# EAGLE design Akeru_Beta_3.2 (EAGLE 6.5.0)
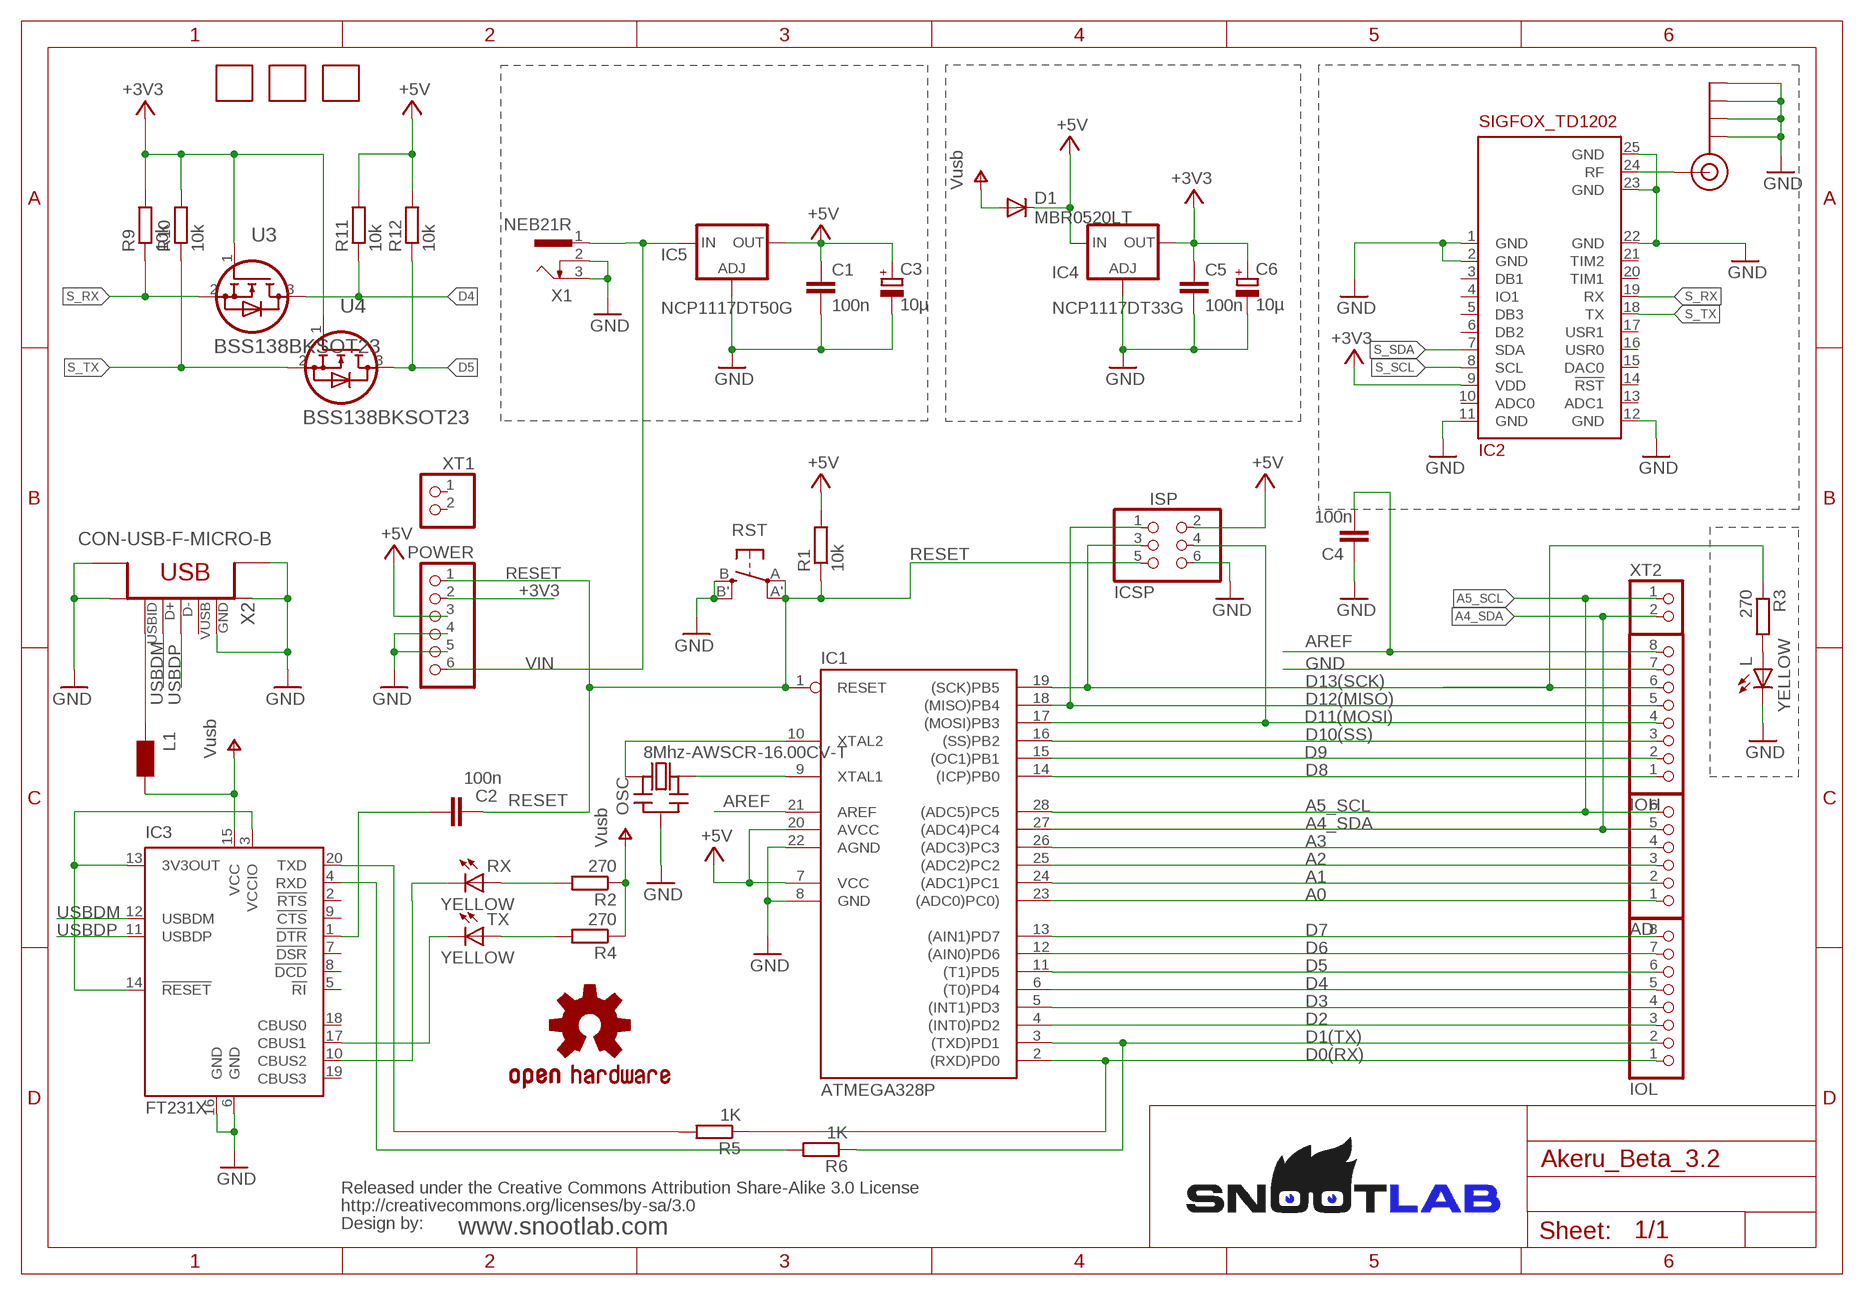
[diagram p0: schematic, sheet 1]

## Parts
AD  PINHD-1X6/STACK  [1X06_STACK]
C1  100n  C-EUC1206  [C1206]
C2  100n  C-EUC1206  [C1206]
C3  10µ  CPOL-EUC  [PANASONIC_C]
C4  100n  C-EUC1206  [C1206]
C5  100n  C-EUC1206  [C1206]
C6  10µ  CPOL-EUC  [PANASONIC_C]
D1  MBR0520LT  [SOD123]
IC1  ATMEGA328P  AT90S4433P  [DIL28-3]
IC2  SIGFOX_TD1202  [TD1202]
IC3  FT231X  [SSOP20]
IC4  NCP1117DT33G  LD117ADT33TR  [DPACK]
IC5  NCP1117DT50G  LD117ADT33TR  [DPACK]
IOH  PINHD-1X8/STACK  [1X08_STACK]
IOL  PINHD-1X8/STACK  [1X08_STACK]
ISP  ICSP  PINHD-2X3  [2X03]
J$1  SMA_EDGE  [SMA_EDGE]
L  YELLOW  LEDCHIPLED_1206  [CHIPLED_1206]
L1  WE-CBF_0805  [0805]
OSC  8Mhz-AWSCR-16.00CV-T  CERMOSCILL-AWCSR  [AWCSR]
POWER  PINHD-1X6/STACK  [1X06_STACK]
R1  10k  R-EU_R1206  [R1206]
R2  270  R-EU_R1206  [R1206]
R3  270  R-EU_R1206  [R1206]
R4  270  R-EU_M1206  [M1206]
R5  1K  R-EU_M1206  [M1206]
R6  1K  R-EU_M1206  [M1206]
R9  10k  R-EU_R1206  [R1206]
R10  10k  R-EU_R1206  [R1206]
R11  10k  R-EU_R1206  [R1206]
R12  10k  R-EU_R1206  [R1206]
RST  SPST_TACT-EVQQ2  [EVQ-Q2]
RX  YELLOW  LEDCHIPLED_1206  [CHIPLED_1206]
TX  YELLOW  LEDCHIPLED_1206  [CHIPLED_1206]
U3  BSS138BKSOT23  [SOT23]
U4  BSS138BKSOT23  [SOT23]
U$1  MARKER  [MARKER]
U$3  CREATIVE_COMMONS  [CREATIVE_COMMONS]
U$4  OSHW-LOGOL  [OSHW-LOGO-L]
U$7  MARKER  [MARKER]
U$8  MARKER  [MARKER]
X1  NEB21R  [NEB21R]
X2  CON-USB-F-MICRO-B  [DX4R005JJ2]
XT1  PINHD-1X2  [1X02_STACK]
XT2  PINHD-1X2  [1X02_STACK]

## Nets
+3V3: C5.1 C6.+ IC2.9(VDD) IC4.4(OUT) POWER.2 R9.2 R10.2 U3.1(G) U4.1(G)
+5V: C1.1 C3.+ D1.C IC1.7(VCC) IC1.20(AVCC) IC4.3(IN) IC5.4(OUT) ISP.2 POWER.3 R1.2 R11.2 R12.2
A0: AD.1 IC1.23((ADC0)PC0))
A1: AD.2 IC1.24((ADC1)PC1)
A2: AD.3 IC1.25((ADC2)PC2)
A3: AD.4 IC1.26((ADC3)PC3)
A4_SDA: AD.5 IC1.27((ADC4)PC4) XT2.2
A5_SCL: AD.6 IC1.28((ADC5)PC5) XT2.1
AREF: C4.2 IC1.21(AREF) IOH.8
D0(RX): IC1.2((RXD)PD0) IOL.1 R5.1
D1(TX): IC1.3((TXD)PD1) IOL.2 R6.1
D2: IC1.4((INT0)PD2) IOL.3
D3: IC1.5((INT1)PD3) IOL.4
D4: IC1.6((T0)PD4) IOL.5 R11.1 U3.3(D)
D5: IC1.11((T1)PD5) IOL.6 R12.1 U4.3(D)
D6: IC1.12((AIN0)PD6) IOL.7
D7: IC1.13((AIN1)PD7) IOL.8
D8: IC1.14((ICP)PB0) IOH.1
D9: IC1.15((OC1)PB1) IOH.2
D10(SS): IC1.16((SS)PB2) IOH.3
D11(MOSI): IC1.17((MOSI)PB3) IOH.4 ISP.4
D12(MISO): IC1.18((MISO)PB4) IOH.5 ISP.1
D13(SCK): IC1.19((SCK)PB5) IOH.6 ISP.3 R3.1
GND: C1.2 C3.- C4.1 C5.2 C6.- IC1.8(GND) IC1.22(AGND) IC2.1(GND) IC2.2(GND) IC2.11(GND) IC2.12(GND) IC2.22(GND) IC2.23(GND) IC2.25(GND) IC3.6(GND) IC3.16(GND) IC4.1(ADJ) IC5.1(ADJ) IOH.7 ISP.6 J$1.GND@0(GND) J$1.GND@1(GND) J$1.GND@2(GND) J$1.GND@3(GND) L.C OSC.2(GND) POWER.4 POWER.5 RST.B'(S1) RST.B(S) X1.2 X1.3 X2.BODY@1(BODY1) X2.BODY@2(BODY2) X2.BODY@3(BODY3) X2.BODY@6(BODY6) X2.P5(GND)
N$1: C2.2 IC3.1(!DTR)
N$2: L.A R3.2
N$3: IC2.24(RF) J$1.SIG(SIGNAL)
N$4: IC3.3(VCCIO) IC3.13(3V3OUT) IC3.14(!RESET)
N$5: IC3.17(CBUS1) TX.C
N$6: L1.1 X2.P4(USBID)
N$9: IC3.10(CBUS2) RX.C
N$10: R2.2 RX.A
N$11: R4.2 TX.A
N$12: IC3.20(TXD) R5.2
N$13: IC3.4(RXD) R6.2
RESET: C2.1 IC1.1(RESET) ISP.5 POWER.1 R1.1 RST.A'(P1) RST.A(P)
S_RX: IC2.19(RX) R9.1 U3.2(S)
S_SCL: IC2.8(SCL)
S_SDA: IC2.7(SDA)
S_TX: IC2.18(TX) R10.1 U4.2(S)
USBDM: IC3.12(USBDM) X2.P3(D+)
USBDP: IC3.11(USBDP) X2.P2(D-)
V+: D1.A IC3.15(VCC) L1.2 R2.1 R4.1 ; supply symbol labelled Vusb
VIN: IC5.3(IN) POWER.6 X1.1
XTAL1: IC1.9(XTAL1) OSC.3(OUT)
XTAL2: IC1.10(XTAL2) OSC.1(IN)
Unconnected: IC2.3(DB1) IC2.4(IO1) IC2.5(DB3) IC2.6(DB2) IC2.10(ADC0) IC2.13(ADC1) IC2.14(!RST) IC2.15(DAC0) IC2.16(USR0) IC2.17(USR1) IC2.20(TIM1) IC2.21(TIM2) IC3.2(!RTS) IC3.5(!RI) IC3.7(!DSR) IC3.8(!DCD) IC3.9(!CTS) IC3.18(CBUS0) IC3.19(CBUS3) X2.P1(VUSB) XT1.1 XT1.2

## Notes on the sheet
- www.snootlab.com

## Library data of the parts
AD POWER = SnootLib:PINHD-1X6: PIN HEADER
C1 C5 = rcl:C-EU: CAPACITOR, European symbol
C2 C4 = SmartPrj:C-EU: CAPACITOR, European symbol
C3 C6 = rcl:CPOL-EU: POLARIZED CAPACITOR, European symbol
D1 = diode:MBR0520LT: SCHOTTKY BARRIER RECTIFIER
IC1 = atmel:AT90S4433: MICROCONTROLLER 4 Kbytes FLASH 128 bytes SRAM 256 bytes EEPROM UART 6-channel 10 bit ADC; OC_FARNELL: unknown; OC_NEWARK: unknown
IC2 = SnootLib:SIGFOX_TD1202: Telecom Design SIGFOX TD1202 - 868MHz
IC3 = ftdichip:FT231X
IC4 IC5 = v-reg:LD117A?*: Low drop fixed and adjustable positive voltage regulators 1 A Source: http://www.st.com/stonline/products/literature/ds/7194/ld1117axx.pdf
IOH IOL = SnootLib:PINHD-1X8: PIN HEADER
ISP = pinhead:PINHD-2X3: PIN HEADER
J$1 = SnootLib:SMA_EDGE: SMA Antenna Connector End launch SMA connector. The paste layer has been removed so that the connector can be hand soldered onto the board after reflow.
L RX TX = led:LED: LED
L1 = wuerth-elektronik:WE-CBF: SMD EMI Suppression Ferrite Beads
OSC = adafruit:CERMOSCILL: Ceramic oscillator with built in capacitors such as ZTT-12MHz http://www.ladyada.net/library/eagle
R1-R6 R9-R12 = rcl:R-EU_: RESISTOR, European symbol
RST = adafruit:SPST_TACT: SMT 6mm switch, EVQQ2 series http://www.ladyada.net/library/eagle
U3 U4 = SnootLib:BSS138BK: N-channel Trench MOSFET
U$1 U$7 U$8 = lib:MARKER
U$3 = SnootLib:CREATIVE_COMMONS
U$4 = SparkFun:OSHW-LOGO: Open Source Hardware Logo This logo indicates the piece of hardware it is found on incorporates a OSHW license and/or adheres to the definition of open source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
X1 = SnootLib:NEB21R: Netzgeräte-Einbaukupplung abgewinkelte Ausführung mit Öffner Source: http://www.lumberg.com/Produkte/PDFs/NEB21R.pdf
X2 = SnootLib:CON-USB-F: USB Female connector
XT1 XT2 = SnootLib:PINHD-1X2

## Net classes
0 default: width 0.254 mm, drill 0.305 mm, clearance 0.152 mm
2 gnd: width 0.305 mm, drill 0.508 mm, clearance 0.152 mm
3 usbvcc: width 0.508 mm, drill 0.508 mm, clearance 0.152 mm

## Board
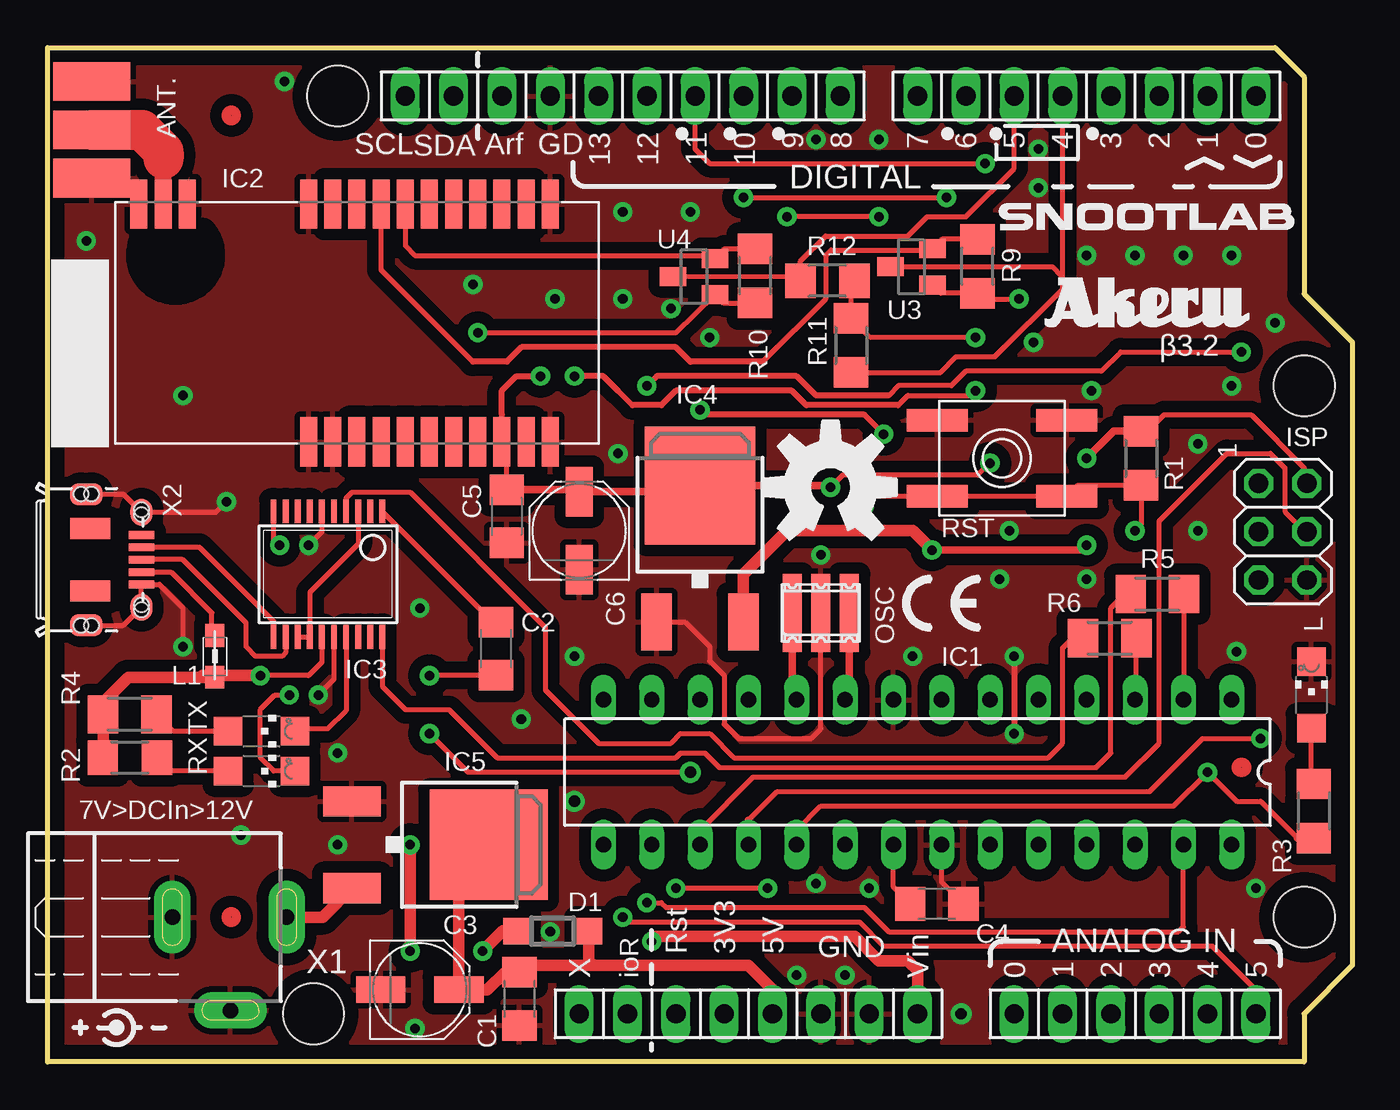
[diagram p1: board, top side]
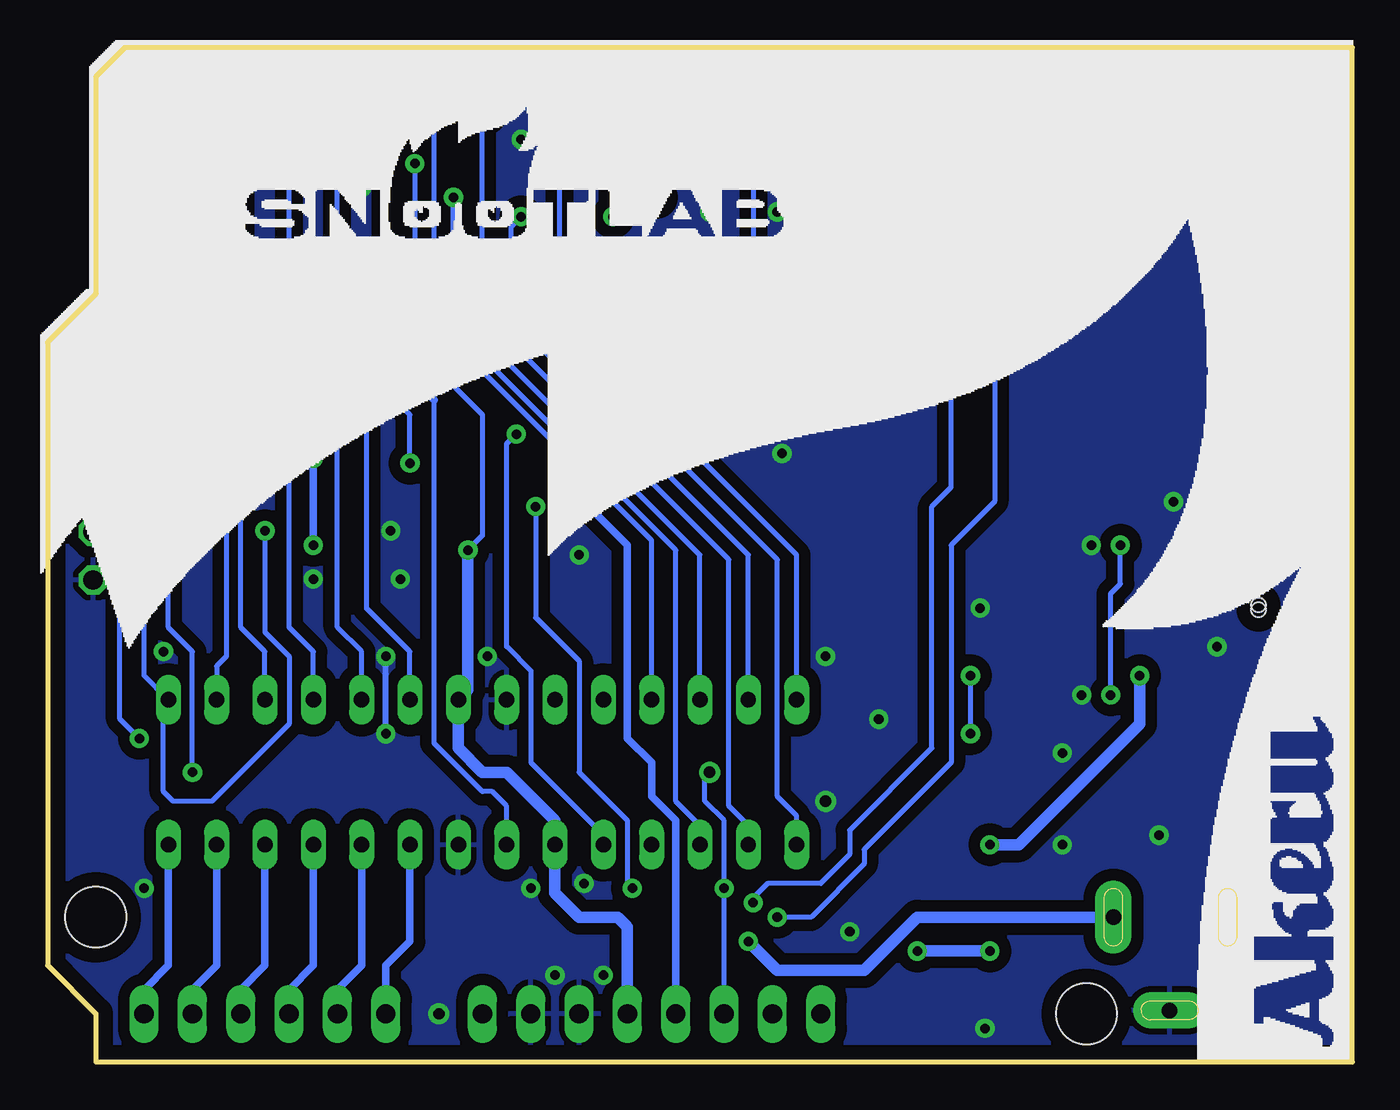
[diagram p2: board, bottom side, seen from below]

Size 68.58 x 53.34 mm. Coordinates in mm from the lower left corner, seen from the top.
Outline: 0,53.34 64.52,53.34 66.04,51.82 66.04,40.39 68.58,37.85 68.58,5.08 66.04,2.54 66.04,0 0,0 0,53.34
Copper layers (1*16): Top 0.035mm / dielectric 1.5mm / Bottom 0.035mm
Design rules "default *": minimum track width 8mil, minimum drill 12mil, track to track 6mil, track to pad 6mil, pad to pad 6mil, via to via 6mil, smd to smd 6mil, copper to edge 30mil, drill to drill 12mil, minimum pad ring 10mil, minimum via ring 10mil, stop-mask expansion 4mil, vias tented up to drill 30mil, thermal gap 12mil
Holes 3.2 mm at 66.04,35.55 66.04,7.61 15.24,50.79 13.97,2.53

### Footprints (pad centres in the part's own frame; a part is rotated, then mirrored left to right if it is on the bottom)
1X06_STACK = drill 1.016 long: 1 -6.35,0; 2 -3.81,0; 3 -1.27,0; 4 1.27,0; 5 3.81,0; 6 6.35,0
C1206 = smd 1.6 x 1.8: 1 -1.4,0; 2 1.4,0
PANASONIC_C = smd 2.6 x 1.4: + 2.05,0; - -2.05,0
SOD123 = smd 1.4 x 1.4: A 1.9,0; C -1.9,0
DIL28-3 = drill 0.813 long: 1 -16.51,-3.81; 2 -13.97,-3.81; 3 -11.43,-3.81; 4 -8.89,-3.81; 5 -6.35,-3.81; 6 -3.81,-3.81; 7 -1.27,-3.81; 8 1.27,-3.81; 9 3.81,-3.81; 10 6.35,-3.81; 11 8.89,-3.81; 12 11.43,-3.81; 13 13.97,-3.81; 14 16.51,-3.81; 15 16.51,3.81; 16 13.97,3.81; 17 11.43,3.81; 18 8.89,3.81; 19 6.35,3.81; 20 3.81,3.81; 21 1.27,3.81; 22 -1.27,3.81; 23 -3.81,3.81; 24 -6.35,3.81; 25 -8.89,3.81; 26 -11.43,3.81; 27 -13.97,3.81; 28 -16.51,3.81
TD1202 = smd 0.89 x 2.6: 1 -2.54,-6.25; 2 -1.27,-6.25; 3 0,-6.25; 4 1.27,-6.25; 5 2.54,-6.25; 6 3.81,-6.25; 7 5.08,-6.25; 8 6.35,-6.25; 9 7.62,-6.25; 10 8.89,-6.25; 11 10.16,-6.25; 12 10.16,6.25; 13 8.89,6.25; 14 7.62,6.25; 15 6.35,6.25; 16 5.08,6.25; 17 3.81,6.25; 18 2.54,6.25; 19 1.27,6.25; 20 0,6.25; 21 -1.27,6.25; 22 -2.54,6.25; 23 -8.92,6.25; 24 -10.19,6.25; 25 -11.46,6.25
SSOP20 = smd 0.305 x 1.245: 1 -2.857,-3.302; 2 -2.222,-3.302; 3 -1.587,-3.302; 4 -0.952,-3.302; 5 -0.317,-3.302; 6 0.318,-3.302; 7 0.953,-3.302; 8 1.588,-3.302; 9 2.223,-3.302; 10 2.858,-3.302; 11 2.858,3.302; 12 2.223,3.302; 13 1.588,3.302; 14 0.953,3.302; 15 0.318,3.302; 16 -0.317,3.302; 17 -0.952,3.302; 18 -1.587,3.302; 19 -2.222,3.302; 20 -2.857,3.302
DPACK = smd 1.6 x 3: 1 -2.28,-4.8; 3 2.28,-4.8 | smd 5.8 x 6.2: 4 0,2.38
1X08_STACK = drill 1.016 long: 1 -8.89,0; 2 -6.35,0; 3 -3.81,0; 4 -1.27,0; 5 1.27,0; 6 3.81,0; 7 6.35,0; 8 8.89,0
2X03 = drill 1.016 octagon: 1 -2.54,-1.27; 2 -2.54,1.27; 3 0,-1.27; 4 0,1.27; 5 2.54,-1.27; 6 2.54,1.27
SMA_EDGE = smd 2.032 x 4.064: GND@0 0,0; GND@1 5.08,0; SIG 2.54,0 | smd 2.032 x 4.064 bottom: GND@2 0,0; GND@3 5.08,0
CHIPLED_1206 = smd 1.5 x 1.5: A 0,-1.75; C 0,1.75
0805 = smd 1.2 x 1: 1 -1.1,0; 2 1.1,0
AWCSR = smd 1 x 4.1: 1 -1.5,0; 2 0,0; 3 1.5,0
R1206 = smd 1.6 x 1.803: 1 -1.422,0; 2 1.422,0
M1206 = smd 1.6 x 2: 1 -1.4,0; 2 1.4,0
EVQ-Q2 = smd 3.2 x 1.2: A -3.4,-2; A' 3.4,-2; B -3.4,2; B' 3.4,2
SOT23 = smd 1 x 1.4: 1 -0.95,-1.1; 2 0.95,-1.1; 3 0,1.1
NEB21R = drill 0.813 pad 1.93 long: 1 0,7.35; 2 4.9,4.4; 3 0,1.35
DX4R005JJ2 = smd 1.4 x 1.15: BODY@1 -2.5,2.9; BODY@2 2.5,2.9 | smd 1.15 x 1.7: BODY@3 3.45,0; BODY@6 -3.45,0 | smd 1.1 x 2.1: BODY@4 1.65,0.2; BODY@5 -1.65,0.2 | smd 0.4 x 1.35: P1 -1.3,2.9; P2 -0.65,2.9; P3 0,2.9; P4 0.65,2.9; P5 1.3,2.9 | hole 0.75: -2.625,2.9; -2.375,2.9; 2.375,2.9; 2.625,2.9; -3.45,0.275; -3.45,-0.275; 3.45,0.275; 3.45,-0.275
1X02_STACK = drill 1.016 long: 1 -1.27,0; 2 1.27,0

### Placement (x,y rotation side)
AD  57.15,2.53 0 top
C1  24.8,3.33 270 top
C2  23.57,21.73 90 top
C3  19.56,3.8 0 top
C4  46.74,8.31 180 top
C5  24.13,28.7 270 top
C6  27.94,27.93 90 top
D1  26.55,6.88 180 top
IC1  45.72,15.23 180 top
IC2  16.26,38.86 0 top
IC3  14.74,25.65 180 top
IC4  34.29,27.93 0 top
IC5  20.8,11.42 270 top
IOH  32.77,50.79 180 top
IOL  54.61,50.79 180 top
ISP  64.91,27.88 270 top
J$1  2.32,46.48 90 top
L  66.42,19.3 0 top
L1  8.8,21.33 270 top
OSC  40.64,23.62 0 top
POWER  39.37,2.53 0 top
R1  57.47,31.74 90 top
R2  4.32,16 0 top
R3  66.55,13.2 90 top
R4  4.32,18.28 0 top
R5  58.33,24.6 180 top
R6  55.82,22.28 180 top
R9  48.87,41.84 270 top
R10  37.18,41.33 270 top
R11  42.23,37.68 90 top
R12  40.99,41.08 0 top
RST  50.17,31.74 0 top
RX  11.24,15.3 270 top
TX  11.24,17.39 270 top
U3  45.41,41.81 90 top
U4  33.98,41.3 90 top
U$1  62.74,15.49 0 top
U$2  [CE3.08X4.13_TOP]  47.76,24.12 0 top
U$3  not placed on the board
U$4  41.15,30.22 0 top
U$5  [LOGO_SNOOT_FULL_H5]  not placed on the board
U$7  9.66,7.61 0 top
U$8  9.66,49.78 0 top
U$9  [LOGO_SNOOT_TXT_H1.7]  49.96,43.66 0 top
X1  5.21,7.61 270 top
X2  2.04,26.41 270 top
XT1  29.21,2.53 0 top
XT2  20.07,50.79 0 top

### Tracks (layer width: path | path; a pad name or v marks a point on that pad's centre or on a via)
+3V3  (via drill 0.5, 0.5 pad 0.25)
  Top 0.254: v22.61,38.35 33,38.35 U4.1 35.52,39.91 R10.2 | v49.53,31.49 48.9,30.85 41.79,30.85 v41.15,30.22 | C5.1 24.13,32.35 IC2.9 23.88,34.03 | U3.1 46.95,40.42 R9.2 49.37,40.13 v51.06,40.13
  Top 0.305: 23.88,34.03 23.88,35.3 24.64,36.06 v25.91,36.06
  Top 0.406: C5.1 27.83,30.1 C6.+ 33.96,29.98 IC4.4 41.06,30.31 v41.15,30.22
  Bottom 0.254: v49.53,31.49 49.53,34.03 50.04,34.54 50.04,39.11 v51.06,40.13
  Bottom 0.305: v25.91,36.06 25.91,36.57 24.13,38.35 v22.61,38.35
  Bottom 0.406: POWER.2 35.56,12.69 36.83,13.96 36.83,15.74 38.1,17.01 38.1,27.17 v41.15,30.22
+5V  (via drill 0.5, 0.5 pad 0.25)
  Top 0.254: R1.2 57.81,33.17 58.68,34.03 63.25,34.03 66.04,31.24 66.04,30.56 ISP.2 | R12.2 42.23,40.89 R11.2 43.24,38.09 v48.77,38.09
  Top 0.406: 57.41,33.23 R1.2 56.04,33.17 v54.61,31.74 | v54.61,27.17 54.36,26.92 v46.49,26.92
  Top 0.61: 28.71,5.07 25.15,5.07 C1.1 24.04,4.73 23.12,3.8 C3.+ 21.61,11.42 IC5.4 | 28.71,5.07 36.83,5.07 38.1,3.8 POWER.3 | IC4.3 36.57,25.64 38.87,27.93 45.47,27.93 v46.49,26.92 | D1.C 28.45,5.33 28.71,5.07
  Bottom 0.254: v48.77,38.09 48.77,37.08 45.72,34.03 45.72,27.68 v46.49,26.92
  Bottom 0.406: v54.61,31.74 v54.61,27.17 54.61,26.92
  Bottom 0.61: POWER.3 38.1,7.11 38.61,7.61 40.64,7.61 41.91,8.88 IC1.20 41.91,12.69 44.45,15.23 45.72,15.23 46.99,16.5 IC1.7 46.49,19.55 v46.49,26.92
A0
  Bottom 0.406: AD.1 50.8,5.07 49.53,6.34 IC1.23
A1
  Bottom 0.406: AD.2 53.34,3.8 52.07,5.07 IC1.24
A2
  Bottom 0.406: AD.3 55.88,3.8 54.61,5.07 IC1.25
A3
  Bottom 0.406: AD.4 58.42,3.8 57.15,5.07 IC1.26
A4_SDA  (via drill 0.5 pad 0.25)
  Top 0.254: v31.5,8.38 32.26,8.38 32.52,8.12 42.93,8.12 44.2,6.85 59.44,6.85 59.69,7.11 IC1.27
  Bottom 0.254: XT2.2 21.09,50.54 21.09,30.22 22.1,29.2 22.1,16.5 26.42,12.19 26.42,10.92 27.94,9.39 30.74,9.39 31.5,8.63 v31.5,8.38
  Bottom 0.406: AD.5 60.96,3.8 59.69,5.07 IC1.27
A5_SCL  (via drill 0.5 pad 0.25)
  Top 0.254: v30.23,7.61 30.48,7.36 42.68,7.36 43.95,6.09 61.22,6.09 63.5,3.8 AD.6
  Bottom 0.254: XT2.1 18.8,29.46 21.09,27.17 21.09,15.74 25.66,11.17 25.66,10.41 28.45,7.61 v30.23,7.61
  Bottom 0.406: IC1.28 62.23,5.07 63.5,3.8 AD.6
AREF  (via drill 0.5 pad 0.25)
  Top 0.254: 29.98,35.3 30.74,34.54 | 44.71,34.54 45.22,35.05 48.52,35.05 v48.77,35.3 | C4.2 44.45,9.2 IC1.21
  Top 0.305: 29.98,35.3 29.21,36.06 v27.69,36.06 | 44.71,34.54 39.88,34.54 39.12,35.3 33.02,35.3 32.26,34.54 30.74,34.54
  Bottom 0.254: 48.26,34.79 48.26,16.76 45.72,14.22 45.22,14.22 44.45,13.46 IC1.21
  Bottom 0.305: v27.69,36.06 23.88,39.87 IOH.8
  Bottom 0.406: v48.77,35.3 48.26,34.79
D0(RX)
  Top 0.254: 59.73,19.14 R5.1
  Top 0.406: IC1.2 59.66,19.08 59.73,19.14
  Bottom 0.254: IOL.1 63.5,40.13 59.19,35.81 59.19,21.33 59.69,20.82 IC1.2
D1(TX)
  Top 0.254: 57.22,19.24 R6.1
  Top 0.406: IC1.3 57.09,19.11 57.22,19.24
  Bottom 0.254: IC1.3 57.15,21.58 58.42,22.85 58.42,36.82 60.96,39.36 IOL.2
D2
  Bottom 0.254: IC1.4 54.61,21.58 55.88,22.85 55.88,36.82 58.42,39.36 IOL.3
D3
  Bottom 0.254: IC1.5 52.07,21.58 53.34,22.85 53.34,36.82 55.88,39.36 IOL.4
D4
  Top 0.254: 53.34,41.4 53.34,40.63 49.79,37.08 47.76,37.08 46.94,36.26 R11.1 | 53.34,41.4 IOL.5 | 53.34,41.4 53.28,41.33 52.8,41.81 U3.3
  Bottom 0.254: IC1.6 49.53,21.58 51.82,23.87 51.82,36.57 53.34,38.09 IOL.5
D5
  Top 0.254: 50.8,47.24 IOL.6 50.8,46.98 48.26,44.44 46.23,44.44 45.22,43.43 40.9,43.43 39.57,42.1 R12.1 39.32,41.33 U4.3
  Bottom 0.254: IC1.11 36.83,27.43 50.8,41.4 IOL.6
D6
  Bottom 0.254: IC1.12 34.29,26.66 48.26,40.63 IOL.7
D7
  Bottom 0.254: IC1.13 31.75,26.66 45.72,40.63 IOL.8
D8
  Bottom 0.254: IOH.1 41.66,46.98 | IC1.14 29.21,26.66 41.66,39.11 41.66,46.73
  Bottom 0.406: 41.66,46.98 41.66,46.73
D9  (via drill 0.5 pad 0.25)
  Top 0.254: v43.69,44.44 v38.87,44.44
  Bottom 0.254: IC1.15 29.21,12.95 30.23,13.96 30.23,26.41 44.2,40.38 44.2,43.94 v43.69,44.44 | v38.87,44.44 38.87,50.54
  Bottom 0.406: 38.87,50.54 IOH.2
D10(SS)  (via drill 0.5 pad 0.25)
  Top 0.254: v36.58,45.46 v47.25,45.46
  Bottom 0.254: IC1.16 31.75,12.44 32.77,13.46 32.77,26.41 47.25,40.89 v47.25,45.46 | v36.58,45.46 IOH.3
D11(MOSI)  (via drill 0.5)
  Top 0.254: 34.29,11.68 34.29,12.19 37.09,14.98 56.65,14.98 58.42,16.76 58.42,28.44 61.98,32 64.27,32 65.03,31.24 65.03,28.95 66.09,27.88 ISP.4 | v49.28,47.24 34.8,47.24 34.04,48 IOH.4
  Top 0.406: IC1.17 34.29,11.68
  Bottom 0.254: IC1.17 34.29,12.44 35.56,13.71 35.56,26.92 49.28,40.63 v49.28,47.24
D12(MISO)  (via drill 0.5, 0.5 pad 0.25)
  Top 0.254: 36.83,12.69 38.36,14.22 57.92,14.22 60.71,17.01 v63.76,17.01 | v62.74,37.33 56.39,37.33 55.38,36.32 48.26,36.32 47.5,35.55 44.71,35.55 44.2,35.05
  Top 0.305: 44.2,35.05 40.39,35.05 39.37,36.06 32.01,36.06 v31.5,35.55
  Top 0.406: IC1.18 36.83,12.69
  Bottom 0.254: IOH.5 v31.5,35.55 | v62.74,37.33 63.25,36.82 63.25,30.82 ISP.1 64.77,29.29 64.77,18.03 v63.76,17.01
D13(SCK)  (via drill 0.5 pad 0.25)
  Top 0.254: 42.93,34.03 v43.95,33.01 | IC1.19 39.37,12.19 40.64,13.46 59.19,13.46 v60.96,15.23 62.49,13.71 63.76,13.71 65.69,11.78
  Top 0.305: 42.93,34.03 34.55,34.03 v34.29,34.28
  Top 0.406: 65.69,11.78 R3.1
  Bottom 0.254: v60.96,15.23 60.96,21.58 62.23,22.85 62.23,27.93 63.59,27.93 ISP.3 | IOH.6 28.96,34.54 | 39.37,11.93 43.18,15.74 43.18,20.57 44.45,21.84 44.45,32.51 v43.95,33.01
  Bottom 0.305: 28.96,34.54 28.96,34.28 29.47,33.78 33.79,33.78 v34.29,34.28
  Bottom 0.406: 39.37,11.93 IC1.19
GND  (via drill 0.5 pad 0.25, 0.6 pad 0.25)
  Top 0.254: 15.05,22.66 IC3.16 15.05,20.12 v14.23,19.3 | IC4.1 33.51,23.13 34.8,21.84 34.8,21.08 35.56,20.31 35.56,17.77 36.33,17.01 40.14,17.01 40.64,17.52 OSC.2 | C4.1 46.99,9.46 IC1.22 | IC3.6 14.42,27.87 v13.72,27.17 | v7.12,21.84 7.12,23.87 5.88,25.11 X2.P5 X2.BODY@2 3.99,22.96 X2.BODY@3 | X2.BODY@6 3.99,29.86 X2.BODY@1 8.85,28.91 v9.4,29.46
  Top 0.305: 50.8,21.08 v50.8,17.27
  Bottom 0.305: v50.8,17.27 v50.8,21.33
  other vias: 27.69,21.33 7.12,35.05 10.16,11.93 26.42,6.85 27.69,13.71 45.47,21.33 50.04,25.39 48.01,2.53 63.5,9.14 64.52,38.86 62.23,35.55 60.46,27.93 32.77,39.62 15.24,16.25 19.31,1.77 50.55,27.93 26.67,40.13 22.36,40.89 60.46,32.51 54.87,35.3 29.98,32 40.64,26.66 39.37,4.57 52.07,48 51.82,37.84 52.07,45.97 54.61,42.41 57.15,42.41 59.69,42.41 41.91,4.57 43.18,9.14 40.39,9.39 34.8,38.09 62.49,21.58 54.61,25.39 62.23,42.41 15.24,11.42 43.69,48.51 40.39,48.51 30.23,44.7 30.23,40.13 33.79,44.7 2.04,43.17 12.45,51.56 24.9,18.03 19.56,23.87
  pour Bottom (isolate 0.61, rank 2): -1.52,52.7 67.69,52.7 67.95,52.44 67.95,0.63 -1.52,0.63
  pour Top (isolate 0.61, rank 2): -1.9,52.7 68.33,52.57 68.33,0.5 -1.9,0.63
N$1
  Top 0.254: IC3.1 23.41,23.13 C2.2
N$2
  Top 0.254: 66.42,14.75 L.A
  Top 0.406: R3.2 66.42,14.75
N$3
  Top 0.9: IC2.24 6.07,47.46 6.1,47.49
  Top 2.1: J$1.SIG 4.96,49.02 6.1,47.87 6.1,47.49
N$4
  Top 0.254: IC3.13 IC3.14 13.78,24.69 16.32,27.23 IC3.3
N$5
  Top 0.254: 13.63,17.52 TX.C 13.12,17.52 14.74,17.52 15.69,18.47 IC3.17
N$6
  Top 0.254: X2.P4 6.5,25.76 8.64,23.62 8.64,22.43 L1.1
N$9  (via drill 0.5)
  Top 0.254: 13.56,14.73 RX.C 11.88,15.3 11.18,16 11.18,18.54 11.94,19.3 v12.7,19.3 | v12.2,27.17 11.88,27.49 IC3.10
  Bottom 0.254: v12.7,19.3 12.7,24.63 12.2,25.14 v12.2,27.17
N$10
  Top 0.254: RX.A 6.44,15.3 R2.2
N$11
  Top 0.254: TX.A 6.61,17.39 R4.2
N$12
  Top 0.254: R5.2 56.61,24.6 55.88,23.87 55.88,16.25 55.12,15.49 35.31,15.49 34.55,16.25 33.28,16.25 33.02,16 23.63,16 21.09,18.54 18.8,18.54 17.59,19.74 IC3.20
N$13
  Top 0.254: 15.69,28.89 IC3.4 15.69,29.65 16.01,29.97 19.05,29.97 26.17,22.85 26.17,19.55 28.96,16.76 32.77,16.76 33.28,17.27 34.8,17.27 36.07,16 52.58,16 53.34,16.76 53.34,21.77 53.85,22.28 R6.2
RESET  (via drill 0.5 pad 0.25, 0.6 pad 0.25)
  Top 0.254: v57.15,27.93 57.47,28.25 R1.1 54.15,30.32 RST.A' RST.A 43.47,29.74 v42.93,29.2 | v33.79,15.23 22.1,15.23 v20.07,17.27 | v37.85,9.14 v33.02,9.14 | C2.1 20.09,20.33 v20.07,20.31
  Bottom 0.254: ISP.5 63.5,25.2 63.5,20.31 IC1.1 62.49,18.79 62.49,14.22 61.98,13.71 59.95,13.71 55.88,17.77 55.88,21.33 57.15,22.6 v57.15,27.93 | POWER.1 v33.02,9.14 33.02,12.69 34.04,13.71 34.04,14.98 v33.79,15.23 | v20.07,17.27 v20.07,20.31 | v42.93,29.2 42.93,23.36 40.64,21.08 40.64,15.23 38.1,12.69 38.1,9.39 v37.85,9.14
S_RX
  Top 0.254: 46.23,42.7 41.19,42.7 40.9,42.41 40.9,40.13 37.6,36.82 | 22.36,36.82 17.53,41.65 IC2.19 | 46.25,42.68 46.23,42.7 | 46.23,42.7 46.54,43.01 46.54,42.79 U3.2 47.01,43.26 R9.1
  Top 0.305: 37.6,36.82 33.79,36.82 33.02,37.59 24.9,37.59 24.13,36.82 22.36,36.82
S_TX
  Top 0.254: IC2.18 18.8,42.92 19.31,42.41 34.91,42.41 U4.2 35.58,42.75 R10.1
USBDM
  Top 0.254: IC3.12 12.51,21.52 12.32,21.33 10.93,21.33 10.42,21.84 10.42,23.11 7.12,26.41 X2.P3
USBDP
  Top 0.254: X2.P2 7.99,27.06 11.88,23.17 IC3.11
V+  (via drill 0.5, 0.5 pad 0.25)
  Top 0.254: IC3.15 14.42,21.01 13.72,20.31 v11.18,20.31
  Top 0.61: v22.86,5.84 23.91,6.88 D1.A | v19.05,11.42 v19.05,5.84 | v11.18,20.31 8.12,20.31 L1.2 4.24,20.23 3.05,19.04 3.05,18.41 R4.1 2.92,16.02 R2.1
  Bottom 0.61: v19.05,5.84 v22.86,5.84 | v19.05,11.42 17.53,11.42 11.18,17.77 v11.18,20.31
VIN  (via drill 0.5 pad 0.25)
  Top 0.61: POWER.6 45.72,4.82 45.22,5.33 43.69,5.33 42.42,6.6 32.01,6.6 v31.75,6.34 | X1.1 14.47,7.61 IC5.3
  Bottom 0.61: v31.75,6.34 30.23,4.82 25.66,4.82 22.86,7.61 X1.1
XTAL1
  Top 0.406: OSC.3 42.14,19.27 IC1.9
XTAL2
  Top 0.406: OSC.1 39.14,19.27 IC1.10

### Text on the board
tPlace: ANT. | SDA | 13 | 12 | 11 | 10 | 9 | 8 | 7 | 6 | 5 | 4 | 3 | 2 | 1 | 0 | SCL | Arf | GD | 1 | 7V>DCIn>12V | Rst | 3V3 | 5V | GND | X | ioR | Vin | 0 | 1 | 2 | 3 | 4 | 5
tNames: DIGITAL | β3.2 | ANALOG IN
tValues: Akeru β3.2 | Sigfox & Snootlab
ReferenceLC: PC2
214bmp: D:/SmartProjects/Snc/a4_bn_logo2.bmp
